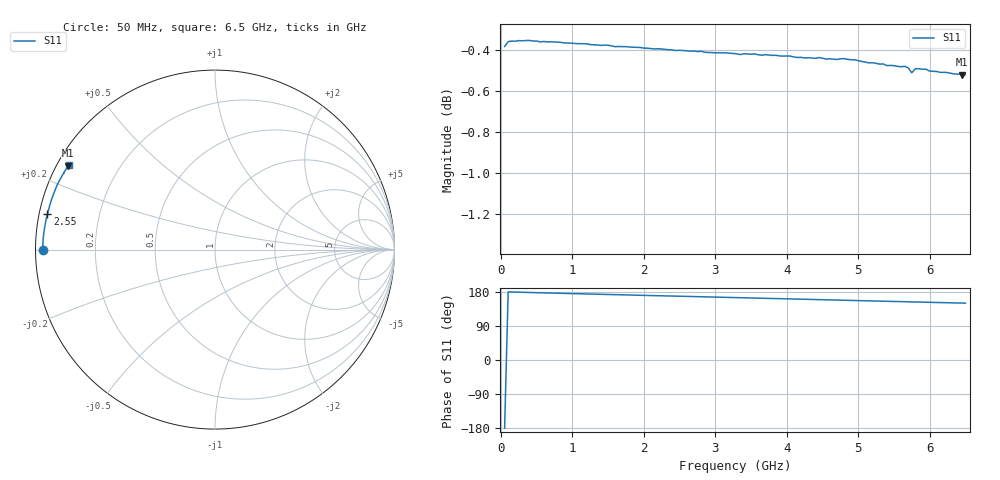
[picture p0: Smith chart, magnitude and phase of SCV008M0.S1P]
! Infineon Technologies  Discrete & RF Semiconductors
! BAR63-02L
! Si PIN Diode in TSLP-2
! IF = 8 mA
! S-Parameters:  March  2002
# GHz  S  MA  R  50
!  f  S11
! GHz  MAG  ANG
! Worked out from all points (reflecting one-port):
!   130 points, 50 MHz to 6.5 GHz, reference 50 ohm
!   lowest |S11| = -0.5 dB at 6.45 GHz (marker M1), VSWR 33.33, Z = 1.61 + j13.3 ohm
!   phase of S11 starts at -180 deg and turns -30 deg over the sweep
!   S11 on the Smith chart (normalised r, x): 50 MHz: 0.02, -0.00; 2.55 GHz: 0.02, +0.11; 6.5 GHz: 0.03, +0.27
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0.05  0.9568 -179.7
0.1  0.9593 179.8
0.25  0.9599 178.9
0.9  0.9586 175.7
1.7  0.9567 172.0
2.05  0.9558 170.3
2.5  0.9547 168.3
2.55  0.9546 168.0
2.7  0.9543 167.4
3.05  0.9534 165.7
3.3  0.9528 164.6
3.4  0.9528 164.2
3.55  0.9528 163.4
3.75  0.9522 162.6
4.1  0.9511 160.9
4.4  0.9504 159.5
4.55  0.95 158.9
4.9  0.9496 157.2
5.15  0.948 156.0
5.3  0.9474 155.4
5.35  0.9474 155.1
5.7  0.9454 153.6
5.75  0.9428 153.1
5.8  0.9449 153.1
5.85  0.9449 152.9
5.9  0.9446 152.6
6.45  0.9417 150.2
6.5  0.9418 150.0
